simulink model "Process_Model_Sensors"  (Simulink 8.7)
settings: Solver=ode45  StartTime=0.0  StopTime=12000  RelTol=1e-3
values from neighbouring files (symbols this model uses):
  Ts = 0.2    [init_model.m]

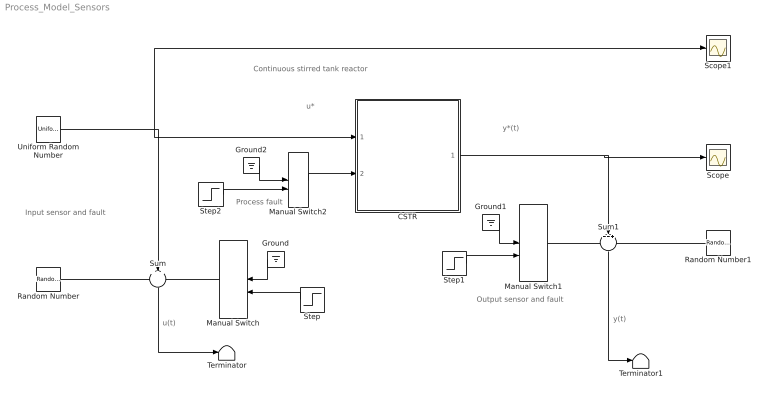
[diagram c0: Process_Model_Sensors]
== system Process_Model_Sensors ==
  note: y(t)
  note: y*(t)
  note: u*
  note: Continuous stirred tank reactor
  note: Process fault
  note: Input sensor and fault
  note: Output sensor and fault
  note: u(t)
  CSTR : Subsystem
  Ground : Ground
  Ground1 : Ground
  Ground2 : Ground
  Manual Switch : ManualSwitch
  Manual Switch1 : ManualSwitch
  Manual Switch2 : ManualSwitch
  Random Number : RandomNumber  Variance=0.0001  Seed=1  SampleTime=Ts
  Random Number1 : RandomNumber  Variance=0.0001  Seed=2  SampleTime=Ts
  Scope : Scope
  Scope1 : Scope
  Step : Step  Time=1000  SampleTime=0
  Step1 : Step  Time=1000  SampleTime=0
  Step2 : Step  Time=1000  SampleTime=0
  Sum : Sum  Inputs=+++  SaturateOnIntegerOverflow=on
  Sum1 : Sum  Inputs=+++  SaturateOnIntegerOverflow=on
  Terminator : Terminator
  Terminator1 : Terminator
  Uniform Random Number : UniformRandomNumber  Minimum=0  Maximum=4  SampleTime=20
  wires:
  Uniform Random Number/1 -> Sum/2, CSTR/1(w), Scope1/1
  Random Number/1 -> Sum/1
  Manual Switch/1 -> Sum/3
  Sum/1 -> Terminator/1
  Ground/1 -> Manual Switch/1
  Step/1 -> Manual Switch/2
  Ground1/1 -> Manual Switch1/1
  Step1/1 -> Manual Switch1/2
  CSTR/1(Cb) -> Sum1/2, Scope/1
  Sum1/1 -> Terminator1/1
  Manual Switch1/1 -> Sum1/1
  Random Number1/1 -> Sum1/3
  Step2/1 -> Manual Switch2/2
  Ground2/1 -> Manual Switch2/1
  Manual Switch2/1 -> CSTR/2(f)

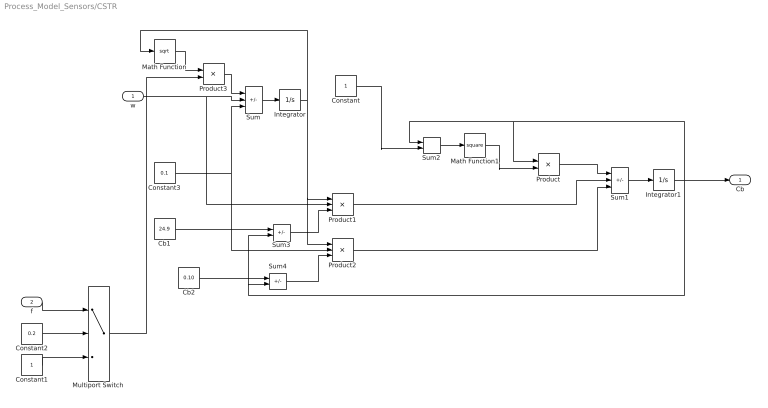
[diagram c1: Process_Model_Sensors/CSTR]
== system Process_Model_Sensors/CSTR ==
  w : Inport
  f : Inport  Port=2
  Cb1 : Constant  Value=24.9
  Cb2 : Constant  Value=0.10
  Constant : Constant
  Constant1 : Constant
  Constant2 : Constant  Value=0.2
  Constant3 : Constant  Value=0.1
  Integrator : Integrator  InitialCondition=30  LimitOutput=on  LowerSaturationLimit=1
  Integrator1 : Integrator  InitialCondition=22
  Math Function : Math  Operator=sqrt
  Math Function1 : Math  Operator=square
  Multiport Switch : MultiPortSwitch  DataPortOrder=Zero-based contiguous  Inputs=2  zeroidx=on
  Product : Product  Inputs=*/  SaturateOnIntegerOverflow=on
  Product1 : Product  Inputs=/**  SaturateOnIntegerOverflow=on
  Product2 : Product  Inputs=/**  SaturateOnIntegerOverflow=on
  Product3 : Product
  Sum : Sum  Inputs=-++  SaturateOnIntegerOverflow=on
  Sum1 : Sum  Inputs=-++  SaturateOnIntegerOverflow=on
  Sum2 : Sum  SaturateOnIntegerOverflow=on
  Sum3 : Sum  Inputs=+-  SaturateOnIntegerOverflow=on
  Sum4 : Sum  Inputs=+-  SaturateOnIntegerOverflow=on
  Cb : Outport
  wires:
  Sum/1 -> Integrator/1
  Product3/1 -> Sum/1
  Math Function/1 -> Product3/1
  Integrator/1 -> Math Function/1, Product1/1, Product2/1
  Sum3/1 -> Product1/3
  Sum4/1 -> Product2/3
  Sum2/1 -> Math Function1/1
  Sum1/1 -> Integrator1/1
  Math Function1/1 -> Product/2
  Product/1 -> Sum1/1
  Product1/1 -> Sum1/2
  Product2/1 -> Sum1/3
  w/1 -> Sum/2, Product1/2
  Constant3/1 -> Product2/2, Sum/3
  Integrator1/1 -> Sum3/2, Sum4/2, Sum2/1, Product/1, Cb/1
  Constant1/1 -> Multiport Switch/3
  f/1 -> Multiport Switch/1
  Constant2/1 -> Multiport Switch/2
  Cb2/1 -> Sum4/1
  Cb1/1 -> Sum3/1
  Constant/1 -> Sum2/2
  Multiport Switch/1 -> Product3/2
